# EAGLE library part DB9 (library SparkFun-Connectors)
DB9 Connector Standard DB9 (D-Sub 9) serial connector. Can be used for CAN bus as well as RS485 and RS232. Footprint production proven. Here is the female version connector we sell at SparkFun: 9 Pin Female Serial Connector - PCB Mount (PRT-00429) This connector has been used on the following SparkFun products: SparkFun RS232 Shifter - SMD (PRT-00449) SparkFun RS232 Shifter SMD (No DB9) (PRT-08780)
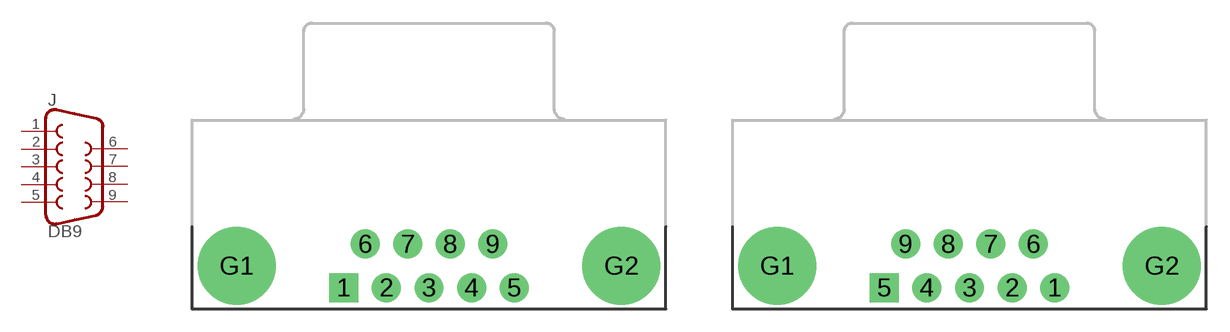
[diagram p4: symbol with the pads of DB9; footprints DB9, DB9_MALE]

Designator prefix J

## DB9FEMALE (PROD_ID: CONN-08194)  [DB9]
1  1  pas
2  2  pas
3  3  pas
4  4  pas
5  5  pas
6  6  pas
7  7  pas
8  8  pas
9  9  pas

## DB9MALE (PROD_ID: CONN-09904)  [DB9_MALE]
Pads as for DB9

## Footprint DB9 (pad centres in mm)
9 Pin Serial Connector - Female PCB Mount Right Angle 0.318" style. Specifications: Pin count:11 Datasheet referenced for footprint Example device(s): DB9
drill 1.016 pad 1.88 square: 1 -5.54,-1.42
drill 1.016 pad 1.88: 2 -2.77,-1.42; 3 0,-1.42; 4 2.77,-1.42; 5 5.54,-1.42; 6 -4.15,1.42; 7 -1.38,1.42; 8 1.38,1.42; 9 4.15,1.42
drill 3.302 pad 5.08: G1 -12.5,0; G2 12.5,0

## Footprint DB9_MALE (pad centres in mm)
9 Pin Serial Connector - Male PCB Mount Right Angle 0.318" style. Specifications: Pin count:11 Datasheet referenced for footprint Example device(s): DB9
drill 1.016 pad 1.88: 1 5.54,-1.42; 2 2.77,-1.42; 3 0,-1.42; 4 -2.77,-1.42; 6 4.15,1.42; 7 1.38,1.42; 8 -1.38,1.42; 9 -4.15,1.42
drill 1.016 pad 1.88 square: 5 -5.54,-1.42
drill 3.302 pad 5.08: G1 -12.5,0; G2 12.5,0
